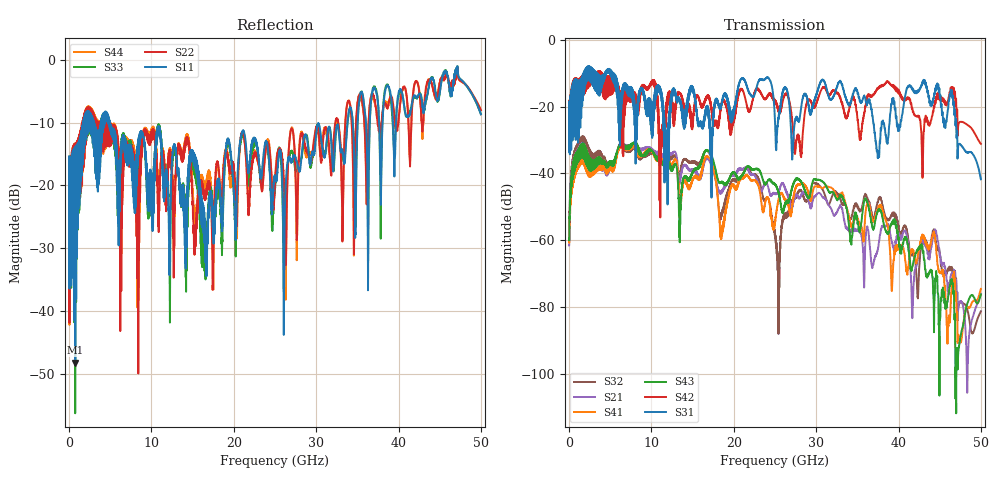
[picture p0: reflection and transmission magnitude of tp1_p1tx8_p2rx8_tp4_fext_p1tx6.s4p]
! 100G CR Analysis
! File: tp1_p1tx8_p2rx8_tp4_fext_p1tx6
! Description: 2m Cu Cable, OSFP, TP1-TP4
! Port Mapping
! Port1 -- P1TX6N
! Port2 -- P2RX8N
! Port3 -- P1TX6P
! Port4 -- P2RX8P
# GHz S MA R 50.00
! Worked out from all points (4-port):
!   5000 points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, 10 MHz to 50 GHz, reference 50 ohm
!   strongest paths, dB at 10 MHz, 12.51 GHz, 25.01 GHz, 37.51 GHz, 50 GHz:
!     S31: -20.7, -15.3, -24.9, -34.9, -41.8
!     S42: -20.5, -17.9, -18.0, -14.7, -31.2
!     S43: -59.6, -39.2, -43.2, -51.4, -76.2
!     S41: -60.2, -37.6, -54.0, -50.5, -74.6
!     S21: -61.6, -34.0, -46.3, -62.5, -76.1
!     S32: -59.8, -35.3, -57.7, -48.4, -81.3
!   lowest |S11| = -48.3 dB at 750 MHz (marker M1), VSWR 1.01, Z = 50.4 - j0.0369 ohm
!   |S11| at or under -10 dB: start of sweep to 1.719 GHz; 3.024 GHz to 3.859 GHz (834.8 MHz wide, 24.3 % of centre); 4.981 GHz to 33.81 GHz (28.83 GHz wide, 149 % of centre)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
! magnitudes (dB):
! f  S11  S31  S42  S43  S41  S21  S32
! 10 MHz  -17.9  -20.7  -20.5  -59.6  -60.2  -61.6  -59.8
! 750 MHz  -48.3  -23.9  -19.2  -36.0  -37.8  -35.8  -33.9
! 21.72 GHz  -17.8  -15.1  -20.8  -37.8  -40.7  -38.8  -38.4
! 25.4 GHz  -16.1  -23.5  -20.5  -45.6  -48.3  -45.9  -68.6
! 37.48 GHz  -6.8  -35.4  -14.6  -51.5  -50.7  -62.7  -48.6
! 43.08 GHz  -7.6  -12.9  -27.3  -65.8  -59.7  -61.2  -59.9
! 50 GHz  -8.7  -41.8  -31.2  -76.2  -74.6  -76.1  -81.3
